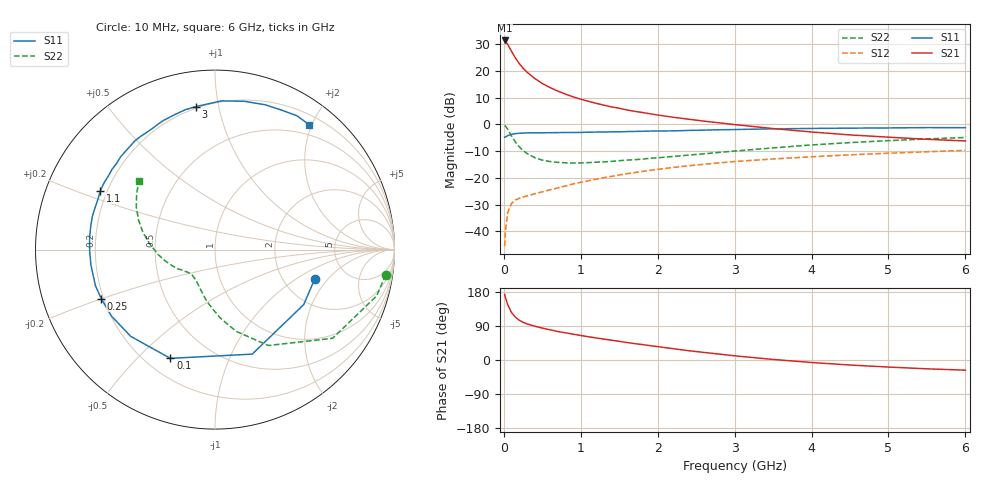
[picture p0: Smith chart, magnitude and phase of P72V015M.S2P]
! SIEMENS Small Signal Semiconductors
! BFP196
! Si NPN RF Bipolar Junction Transistor in SOT143
! VCE = 2 V  IC = 15 mA
! Common Emitter S-Parameters:  May  1996
# GHz  S  MA  R  50
!  f  S11  S21  S12  S22
! GHz  MAG  ANG  MAG  ANG  MAG  ANG  MAG  ANG
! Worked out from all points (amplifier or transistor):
!   36 points, 10 MHz to 6 GHz, reference 50 ohm
!   highest |S21| = 31.4 dB at 10 MHz (marker M1)
!   |S21| within 3 dB of that: start of sweep to 79.94 MHz
!   unconditionally stable (mu >= 1): 722.5 MHz to 3.353 GHz
!   at 250 MHz: K = 0.52, MSG = 24.1 dB, |S12| = -27.1 dB
!   at 1.4 GHz: K = 1.14, MAG = 10.8 dB, |S12| = -19.4 dB
!   at 6 GHz: K = 0.98, MSG = 1.8 dB, |S12| = -9.7 dB
!   S11 on the Smith chart (normalised r, x): 10 MHz: 2.95, -1.47; 100 MHz: 0.30, -0.63; 250 MHz: 0.19, -0.20; 1.1 GHz: 0.17, +0.24; 3 GHz: 0.19, +0.86; 6 GHz: 0.34, +1.96
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0.01  0.5792 -16.6  37.26 173.2  0.0053 81.8  0.9615 -8.4
0.02  0.5816 -31.8  35.88 165.0  0.01 76.4  0.9366 -16.0
0.05  0.6181 -70.4  31.61 146.3  0.0225 62.1  0.8208 -37.0
0.1  0.655 -112.3  23.37 125.2  0.0334 46.2  0.6116 -60.9
0.15  0.6739 -134.2  17.5 112.9  0.0387 39.7  0.4695 -75.6
0.2  0.6854 -147.3  13.85 105.0  0.0416 37.4  0.3827 -85.5
0.25  0.6903 -156.7  11.28 99.4  0.0441 37.2  0.3238 -93.4
0.3  0.6958 -163.2  9.55 95.4  0.046 37.2  0.2883 -99.5
0.4  0.6966 -173.0  7.287 89.3  0.0505 39.6  0.2404 -109.0
0.5  0.6986 -179.6  5.846 84.2  0.055 41.7  0.2154 -115.9
0.6  0.702 174.5  4.899 79.6  0.06 43.9  0.2027 -121.5
0.7  0.7046 169.0  4.224 75.2  0.065 45.5  0.1956 -126.1
0.9  0.708 160.7  3.287 68.2  0.0772 47.7  0.1899 -132.6
1.1  0.7182 152.8  2.708 61.4  0.0886 48.7  0.1938 -137.2
1.3  0.722 145.2  2.297 55.1  0.1011 48.8  0.1999 -141.7
1.6  0.7372 135.5  1.87 46.1  0.1199 47.8  0.2157 -147.5
2.2  0.7589 117.8  1.366 29.9  0.157 43.1  0.2523 -158.5
3  0.8038 97.7  0.995 11.0  0.2027 34.2  0.3183 -175.1
3.5  0.8295 87.5  0.839 1.5  0.2266 28.3  0.3648 175.1
4.5  0.8541 70.8  0.638 -13.3  0.2708 17.1  0.4581 158.6
5.5  0.8744 58.4  0.528 -23.3  0.3092 6.2  0.5371 144.4
6  0.8712 52.9  0.492 -26.8  0.3273 0.2  0.5713 137.8
